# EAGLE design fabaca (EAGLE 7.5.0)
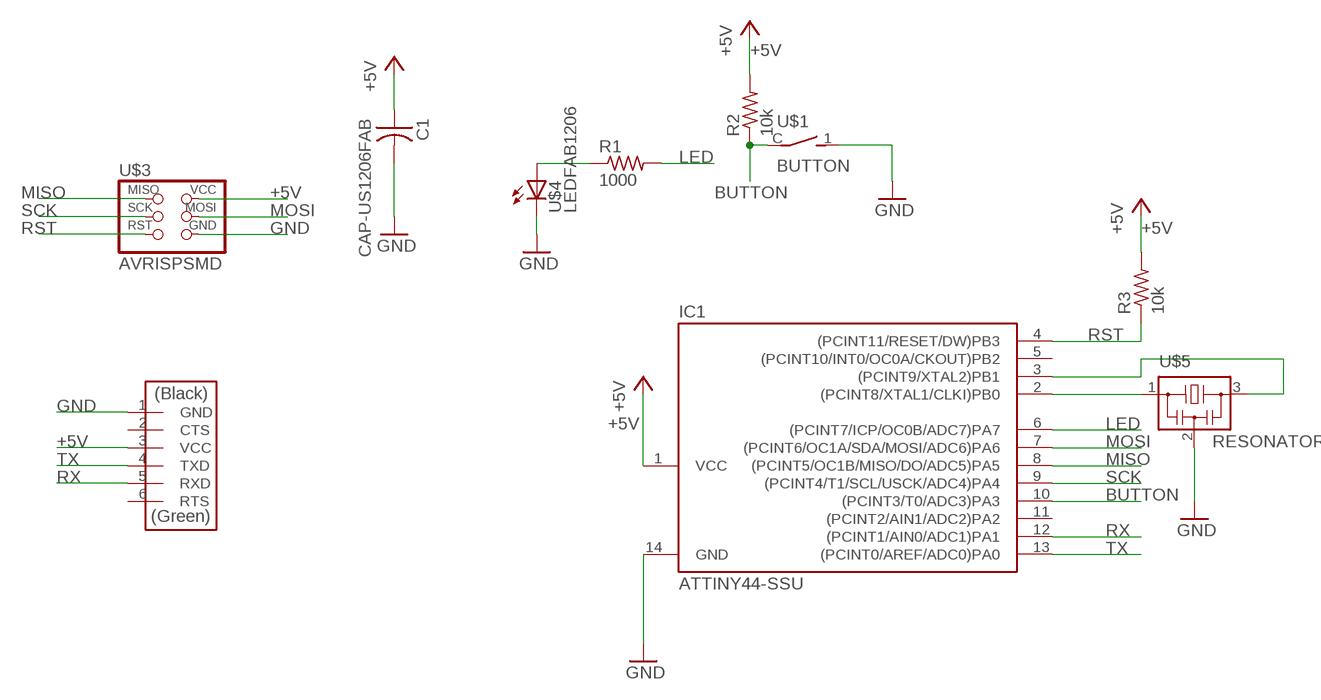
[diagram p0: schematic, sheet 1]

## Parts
C1  CAP-US1206FAB  [C1206FAB]
IC1  ATTINY44-SSU  [SOIC14]
R1  1000  RES-US1206FAB  [R1206FAB]
R2  10k  RES-US1206FAB  [R1206FAB]
R3  10k  RES-US1206FAB  [R1206FAB]
U$1  BUTTON  [BUT-NPS]
U$2  FTDI-SMD-HEADER  [1X06SMD]
U$3  AVRISPSMD  [2X03SMD]
U$4  LEDFAB1206  [LED1206FAB]
U$5  RESONATOR  [EFOBM]

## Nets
+5V: C1.1 IC1.1(VCC) R2.2 R3.2 U$2.3(VCC) U$3.2(VCC)
BUTTON: IC1.10((PCINT3/T0/ADC3)PA3) R2.1 U$1.C
GND: C1.2 IC1.14(GND) U$1.1 U$2.1(GND) U$3.6(GND) U$4.2(C) U$5.2
LED: IC1.6((PCINT7/ICP/OC0B/ADC7)PA7) R1.2
MISO: IC1.8((PCINT5/OC1B/MISO/DO/ADC5)PA5) U$3.1(MISO)
MOSI: IC1.7((PCINT6/OC1A/SDA/MOSI/ADC6)PA6) U$3.4(MOSI)
N$1: IC1.3((PCINT9/XTAL2)PB1) U$5.3
N$2: IC1.2((PCINT8/XTAL1/CLKI)PB0) U$5.1
N$11: R1.1 U$4.1(A)
RST: IC1.4((PCINT11/RESET/DW)PB3) R3.1 U$3.5(RST)
RX: IC1.12((PCINT1/AIN0/ADC1)PA1) U$2.5(RXD)
SCK: IC1.9((PCINT4/T1/SCL/USCK/ADC4)PA4) U$3.3(SCK)
TX: IC1.13((PCINT0/AREF/ADC0)PA0) U$2.4(TXD)
Unconnected: IC1.5((PCINT10/INT0/OC0A/CKOUT)PB2) IC1.11((PCINT2/AIN1/ADC2)PA2) U$2.2(CTS) U$2.6(RTS)

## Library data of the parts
C1 = HelloKamakura:CAP-US
IC1 = HelloKamakura:ATTINY44
R1-R3 = HelloKamakura:RES-US: Resistor (US Symbol)
U$1 = HelloKamakura:BUTTON: Distribute : Akizuki Densi
U$2 = HelloKamakura:FTDI-SMD-HEADER
U$3 = HelloKamakura:AVRISP
U$4 = HelloKamakura:LED: LED
U$5 = HelloKamakura:RESONATOR

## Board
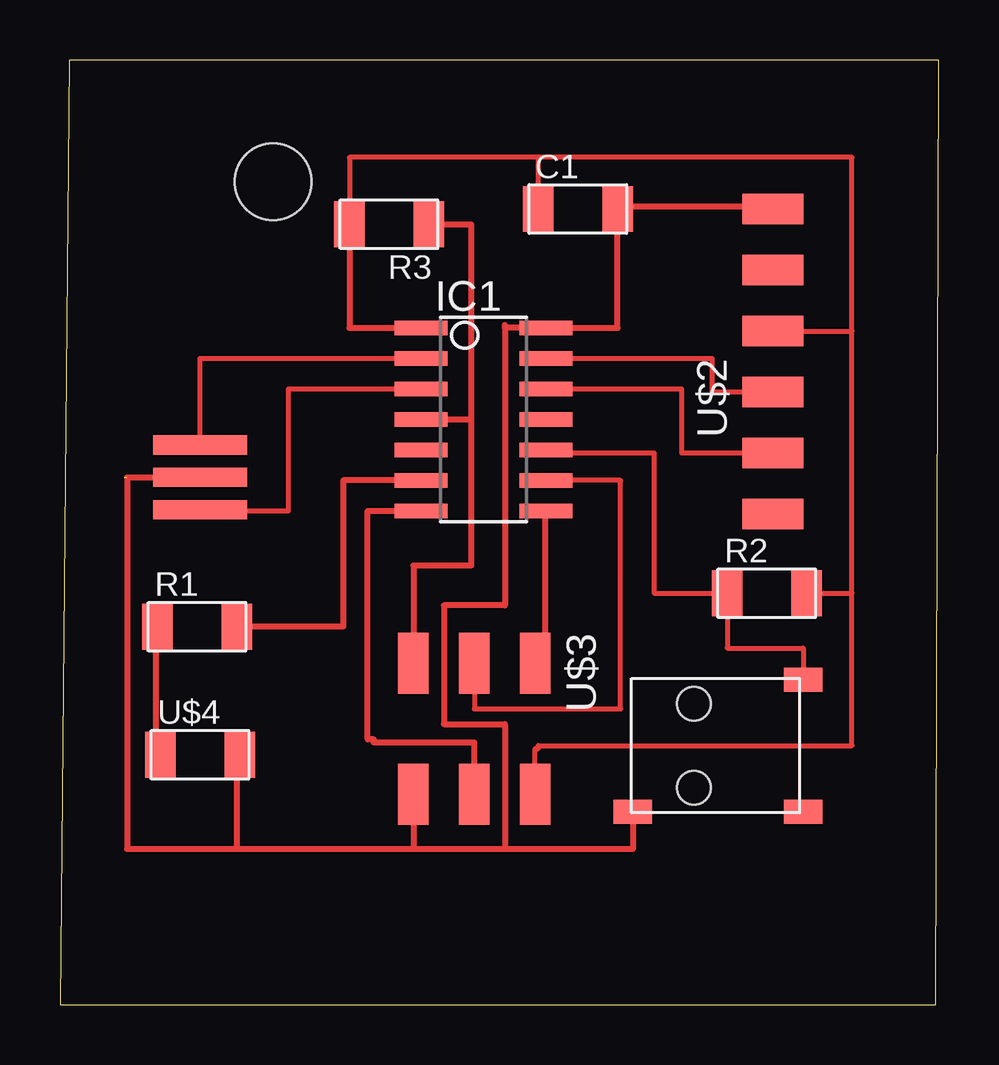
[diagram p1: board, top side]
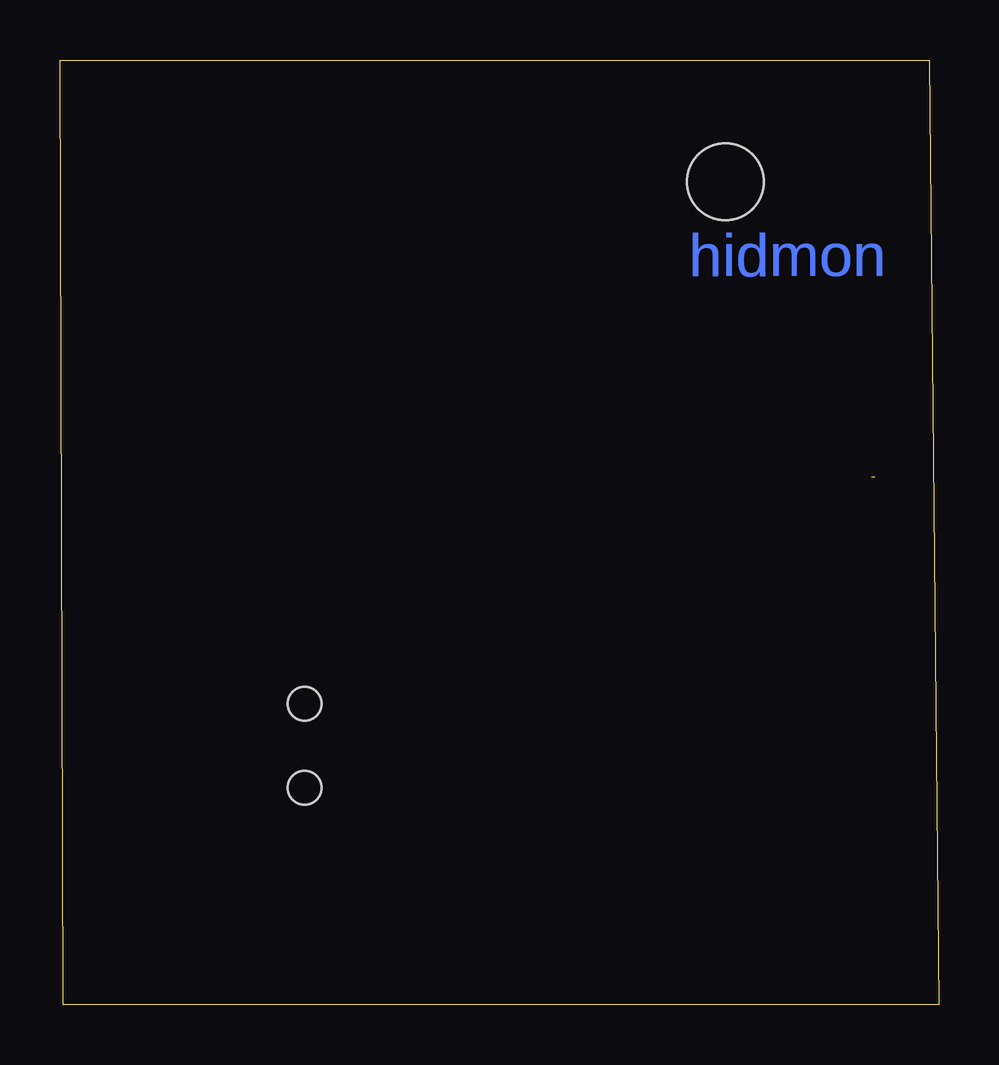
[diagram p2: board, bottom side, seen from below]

Size 36.63 x 39.36 mm. Coordinates in mm from the lower left corner, seen from the top.
Outline: 0,0 36.5,0 36.63,39.36 0.38,39.36 0,0
Copper layers (1*16): Top 0.035mm / dielectric 1.5mm / Bottom 0.035mm
Design rules "default": minimum track width 10mil, minimum drill 24mil, track to track 8mil, track to pad 8mil, pad to pad 8mil, via to via 8mil, smd to smd 8mil, copper to edge 40mil, drill to drill 8mil, minimum pad ring 10mil, minimum via ring 8mil, stop-mask expansion 4mil, vias tented up to drill 0mil, thermal gap 10mil
Holes 3.2 mm at 8.89,34.29

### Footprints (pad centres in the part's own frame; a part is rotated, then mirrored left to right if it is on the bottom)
C1206FAB = smd 1.27 x 1.905: 1 -1.651,0; 2 1.651,0
SOIC14 = smd 0.61 x 2.21: 1 -3.81,-2.603; 2 -2.54,-2.603; 3 -1.27,-2.603; 4 0,-2.603; 5 1.27,-2.603; 6 2.54,-2.603; 7 3.81,-2.603; 8 3.81,2.603; 9 2.54,2.603; 10 1.27,2.603; 11 0,2.603; 12 -1.27,2.603; 13 -2.54,2.603; 14 -3.81,2.603
R1206FAB = smd 1.27 x 1.905: 1 -1.651,0; 2 1.651,0
BUT-NPS = smd 1 x 1.6: 1 2.75,-3.55; C -2.75,3.55; P$1 2.75,3.55 | hole 1.4: -1.75,-1; 1.75,-1
1X06SMD = smd 2.54 x 1.27: 1 0,6.35; 2 0,3.81; 3 0,1.27; 4 0,-1.27; 5 0,-3.81; 6 0,-6.35
2X03SMD = smd 2.54 x 1.27: 1 -2.54,2.54; 2 2.92,2.54; 3 -2.54,0; 4 2.92,0; 5 -2.54,-2.54; 6 2.92,-2.54
LED1206FAB = smd 1.27 x 1.905: 1 -1.651,0; 2 1.651,0
EFOBM = smd 0.8 x 3.9: 1 -1.35,0; 2 0,0; 3 1.35,0

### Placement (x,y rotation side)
C1  21.59,33.15 0 top
IC1  17.65,24.38 270 top
R1  5.71,15.75 0 top
R2  29.46,17.14 0 top
R3  13.72,32.51 180 top
U$1  27.43,10.79 270 top
U$2  29.72,26.8 0 top
U$3  17.27,11.68 270 top
U$4  5.84,10.41 0 top
U$5  5.84,21.97 270 top

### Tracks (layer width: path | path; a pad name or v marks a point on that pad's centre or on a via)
+5V
  Top 0.203: U$3.2 19.81,10.67 19.94,10.67 19.94,10.79 33.02,10.79 33.02,17.14 | 33.02,17.14 33.02,28.07 | 33.02,28.07 33.02,35.31 19.94,35.31 | 19.94,35.31 12.06,35.31 R3.2 | C1.1 19.94,35.31 | U$2.3 33.02,28.07 | R2.2 33.02,17.14
  Top 0.254: R3.2 12.06,28.19 IC1.1
BUTTON
  Top 0.203: IC1.10 20.26,22.99 24.77,22.99 24.77,17.14 R2.1 27.81,14.86 30.99,14.86 U$1.C
GND  (1 unrouted)
  Top 0.254: U$2.1 29.62,33.25 23.44,33.25 C1.2 23.24,28.19 IC1.14 18.54,28.19 | U$1.1 23.88,6.48 18.54,6.48 | 18.54,6.48 14.73,6.48 | 14.73,6.48 7.37,6.48 | 7.37,6.48 2.79,6.48 2.79,21.97 U$5.2 | U$4.2 7.37,10.41 7.37,6.48 | U$3.6 14.73,6.48 | 18.54,28.19 18.54,28.32 | 18.54,28.19 18.54,16.64 16,16.64 16,11.68 18.54,11.68 18.54,6.48
LED
  Top 0.254: IC1.6 11.81,21.84 11.81,15.75 R1.2
MISO
  Top 0.254: IC1.8 20.24,20.45 20.24,14.5 20.02,14.28 U$3.1
MOSI
  Top 0.254: U$3.4 17.27,10.92 13.08,10.92 13.08,11.05 12.83,11.05 12.83,20.57 IC1.7
N$1
  Top 0.203: U$5.3 5.84,20.57 9.53,20.57 9.53,25.65 IC1.3
N$2
  Top 0.203: U$5.1 5.84,26.92 IC1.2
N$11
  Top 0.254: R1.1 4.01,15.65 4.01,10.62 U$4.1
RST
  Top 0.254: 17.14,24.38 17.14,32.51 R3.1 | 17.14,24.38 17.14,18.29 14.73,18.29 U$3.5 | IC1.4 17.14,24.38
RX
  Top 0.203: IC1.12 25.91,25.65 25.91,22.99 U$2.5
SCK
  Top 0.203: U$3.3 17.27,12.32 23.37,12.32 23.37,21.84 IC1.9
TX
  Top 0.203: IC1.13 27.18,26.92 27.18,25.53 U$2.4

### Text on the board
Bottom: hidmon | hidmon | hidmon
